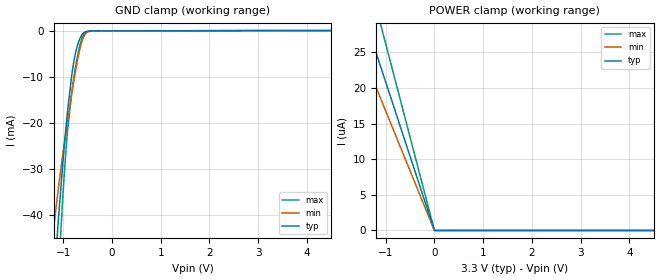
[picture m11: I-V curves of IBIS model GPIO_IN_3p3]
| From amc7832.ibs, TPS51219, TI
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|   Model
[Model]   GPIO_IN_3p3
Model_type   Input
Vinl = 0.99
Vinh = 2.31
|   typ   min   max
C_comp   1pF   1pF   1pF
[Voltage Range]   3.3   3.29   3.31
[Temperature Range]   27   125   -40
[Power Clamp Reference]   3.3   3.29   3.31
[GND Clamp Reference]   -0   -0   -0
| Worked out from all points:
|   GND clamp passes 1 mA (typ) near -0.62 V on its own axis
[GND Clamp]
|   Voltage   I(typ)   I(min)   I(max)
-3.3V     -419.4mA   -290.4mA   -554.8mA
-1.211V   -57.12mA   -44.13mA   -76.4mA
-1.122V   -44.1mA    -36.1mA    -57.77mA
-1.092V   -39.92mA   -33.53mA   -51.78mA
-1.023V   -30.58mA   -27.82mA   -38.54mA
-943.8mV  -20.89mA   -21.87mA   -25.74mA
-914.1mV  -17.66mA   -19.76mA   -21.91mA
-825mV    -9.587mA   -13.65mA   -13.21mA
-706.2mV  -3.125mA   -6.339mA   -5.466mA
-627mV    -1.102mA   -2.723mA   -1.994mA
-547.8mV  -291.1uA   -756.8uA   -447.4uA
6.59V     0A         0A         0A
[POWER Clamp]
|   Voltage   I(typ)   I(min)   I(max)
-3.3V     68.73uA    55.4uA     86.42uA
-1.884V   39.21uA    31.59uA    49.32uA
-1.637V   34.06uA    27.44uA    42.83uA
-1.35V    28.08uA    22.62uA    35.32uA
-1.073V   22.3uA     17.96uA    28.06uA
-3.3mV    31.46nA    11.05nA    56.78nA
6.59V     0A         0A         0A
